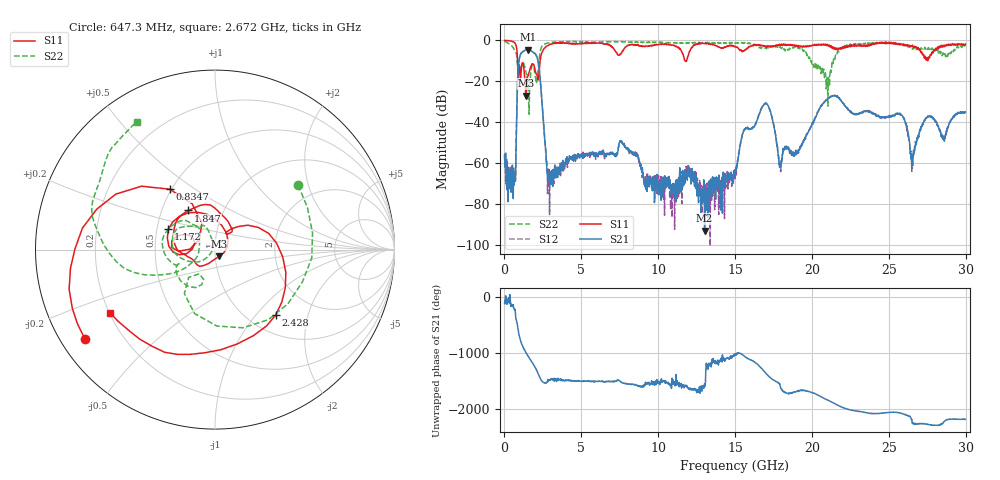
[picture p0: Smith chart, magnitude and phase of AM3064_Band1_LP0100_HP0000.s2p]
# Hz S DB R 50.0
!freq dBS11 angS11 dBS21 angS21 dBS12 angS12 dBS22 angS22
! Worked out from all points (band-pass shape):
!   1600 points, 10 MHz to 29.98 GHz, reference 50 ohm
!   highest |S21| = -4.47 dB at 1.528 GHz (marker M1); lowest = -93.0 dB at 13.02 GHz (marker M2)
!   |S21| within 3 dB of the highest: 1.015 GHz to 2.073 GHz (1.058 GHz wide, 68.5 % of centre)
!   lowest |S11| = -27.0 dB at 1.397 GHz (marker M3), VSWR 1.09, Z = 52.2 - j4 ohm
!   |S11| at or under -10 dB: 848.6 MHz to 2.318 GHz (1.469 GHz wide, 92.8 % of centre); 11.75 GHz to 11.84 GHz (90.84 MHz wide, 0.77 % of centre)
!   |S22| runs from -36.1 to -0.4 dB; largest |S21 - S12| = 0.0083
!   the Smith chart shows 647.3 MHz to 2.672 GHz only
!   S11 on the Smith chart (normalised r, x): 647.3 MHz: 0.07, -0.31; 834.7 MHz: 0.49, +0.40; 1.172 GHz: 0.57, +0.14; 1.847 GHz: 0.68, +0.32; 2.428 GHz: 1.32, -1.28; 2.672 GHz: 0.20, -0.27
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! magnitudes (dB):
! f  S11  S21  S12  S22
! 10 MHz  0.0  -56.1  -56.1  -0.4
! 647.3 MHz  -1.1  -64.4  -65.1  -4.6
! 834.7 MHz  -7.5  -24.8  -24.8  -10.5
! 1.172 GHz  -11.0  -5.7  -5.6  -10.7
! 1.397 GHz  -27.0  -4.5  -4.5  -15.8
! 1.528 GHz  -17.5  -4.5  -4.4  -21.4
! 1.847 GHz  -11.5  -5.7  -5.6  -12.1
! 2.428 GHz  -6.1  -28.9  -28.9  -3.0
! 2.672 GHz  -3.3  -52.4  -53.1  -1.6
! 2.99 GHz  -1.9  -69.5  -66.0  -1.1
! 5.015 GHz  -1.5  -56.1  -56.4  -0.7
! 7.62 GHz  -5.9  -49.9  -49.7  -0.7
! 10 GHz  -2.0  -72.9  -75.9  -0.9
! 13.02 GHz  -1.5  -93.0  -80.8  -1.1
! 15 GHz  -3.1  -63.7  -67.6  -1.4
! 16.92 GHz  -2.8  -31.0  -30.9  -3.8
! 17.95 GHz  -2.4  -61.8  -60.6  -3.3
! 19.99 GHz  -2.7  -41.3  -41.2  -11.1
! 21.42 GHz  -3.9  -27.0  -27.0  -8.7
! 25 GHz  -1.0  -37.6  -37.1  -1.1
! 26.53 GHz  -2.5  -58.6  -57.2  -4.3
! 29.98 GHz  -1.8  -35.0  -35.6  -2.9
